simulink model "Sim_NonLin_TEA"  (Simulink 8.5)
settings: Solver=ode113  StartTime=0.0  StopTime=97200  RelTol=1e-3
InitFcn:
  | start
StopFcn:
  | Pl3
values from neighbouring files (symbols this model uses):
  Ave = [    [vehicle_flex34.m]    (also in vehicle_rigid.m)
  Bve = [    [vehicle_flex34.m]    (also in vehicle_rigid.m)
  CB2L = [cpsi, -cphi*spsi,  sphi*spsi;          0,    cphi,      -sphi;          0,    sphi*cpsi,  cphi*cpsi]/cpsi    [Rigbod_Dynam_LVLH.m]    (also in start.m = eye(3); start2.m = eye(3); start3.m = eye(3); start1.m = eye(3))
  Cve = [    [vehicle_flex34.m]    (also in vehicle_rigid.m)
  Dve = [    [vehicle_flex34.m]    (also in vehicle_rigid.m)
  ini = [wbo; atto; Hco]    [start.m]    (also in start2.m; start3.m; start1.m)
  Kpqr = lqr(sys,Q0,R0)    [des.m]
  nt = 12    [start.m]    (also in start2.m; start3.m; start1.m)
  wo = 0.0011    [start.m]    (also in start2.m; start3.m; start1.m)
undefined symbols (not defined in the file or in its folder): Rigbod_Dynam_LVLH

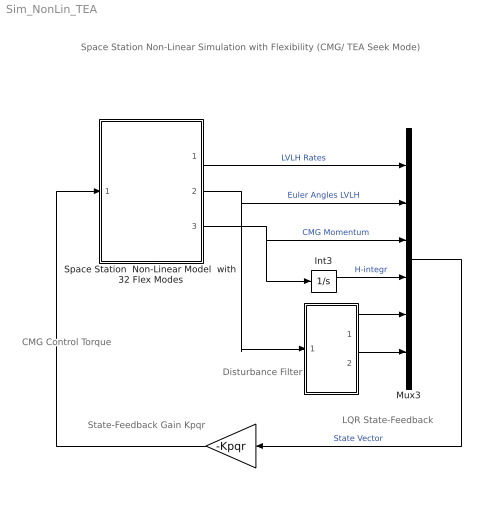
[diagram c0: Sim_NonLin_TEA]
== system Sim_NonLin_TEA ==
  note: Space Station Non-Linear Simulation with Flexibility (CMG/ TEA Seek Mode)
  note: LQR State-Feedback
  note: CMG Control Torque
  note: Disturbance Filter
  note: State-Feedback Gain Kpqr
  " " : Subsystem
  "  " : Gain  Gain=-Kpqr  Multiplication=Matrix(K*u)
  Int3 : Integrator
  Mux3 : Mux  Inputs=[3, 3, 3, 3, 1, 1]
  Space Station  Non-Linear Model  with 32 Flex Modes : Subsystem
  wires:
  Int3/1 -> Mux3/4  "H-integr"
  Space Station  Non-Linear Model  with 32 Flex Modes/3(Hcmg) -> Int3/1, Mux3/3  "CMG Momentum"
  Space Station  Non-Linear Model  with 32 Flex Modes/2(attit-lv) -> Mux3/2, " "/1(the)  "Euler Angles LVLH"
  "  "/1 -> Space Station  Non-Linear Model  with 32 Flex Modes/1(Tcmg)
  Mux3/1 -> "  "/1  "State Vector"
  " "/1(a1) -> Mux3/5
  " "/2(a2) -> Mux3/6
  Space Station  Non-Linear Model  with 32 Flex Modes/1(w-lv) -> Mux3/1  "LVLH Rates"

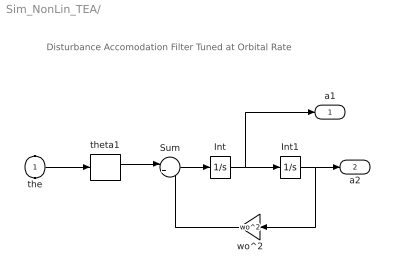
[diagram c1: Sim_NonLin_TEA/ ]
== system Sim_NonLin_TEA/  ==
  note: Disturbance Accomodation Filter Tuned at Orbital Rate
  the : Inport
  Int : Integrator
  Int1 : Integrator
  Sum : Sum  Inputs=|+-
  theta1 : Selector  InputPortWidth=3  Indices=[2]
  wo^2 : Gain  Gain=wo^2
  a1 : Outport
  a2 : Outport  Port=2
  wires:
  Int/1 -> Int1/1, a1/1
  Sum/1 -> Int/1
  Int1/1 -> wo^2/1, a2/1
  wo^2/1 -> Sum/2
  theta1/1 -> Sum/1
  the/1 -> theta1/1

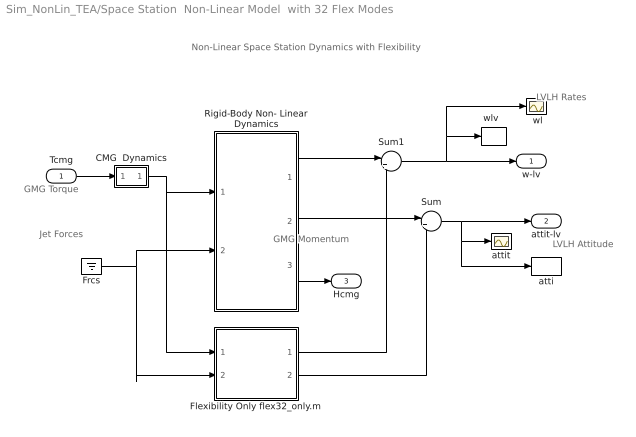
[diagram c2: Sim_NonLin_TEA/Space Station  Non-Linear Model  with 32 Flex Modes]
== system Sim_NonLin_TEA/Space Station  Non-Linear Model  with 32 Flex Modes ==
  note: Non-Linear Space Station Dynamics with Flexibility
  note: GMG Torque
  note: Jet Forces
  note: LVLH Rates
  note: LVLH Attitude
  note: GMG Momentum
  Tcmg : Inport
  " attit " : Scope
  " wl" : Scope
  CMG  Dynamics : Subsystem
  Flexibility Only flex32_only.m : Subsystem
  Frcs : Ground
  Rigid-Body Non- Linear Dynamics : Subsystem
  Sum : Sum  Inputs=|++
  Sum1 : Sum  Inputs=|++
  atti : ToWorkspace  VariableName=theta  SampleTime=-1
  "wlv  " : ToWorkspace  VariableName=wl  SampleTime=-1
  w-lv : Outport
  attit-lv : Outport  Port=2
  Hcmg : Outport  Port=3
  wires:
  Frcs/1 -> Rigid-Body Non- Linear Dynamics/2(Frcs), Flexibility Only flex32_only.m/2(Frcs)
  Rigid-Body Non- Linear Dynamics/2(atti-lv) -> Sum/1
  Flexibility Only flex32_only.m/2(att) -> Sum/2
  Sum/1 -> attit-lv/1, " attit "/1, atti/1
  Sum1/1 -> w-lv/1, "wlv  "/1, " wl"/1
  Tcmg/1 -> CMG  Dynamics/1(I)
  Rigid-Body Non- Linear Dynamics/1(w-lv) -> Sum1/1
  Flexibility Only flex32_only.m/1(wbf) -> Sum1/2
  Rigid-Body Non- Linear Dynamics/3(Hcmg) -> Hcmg/1
  CMG  Dynamics/1(O) -> Rigid-Body Non- Linear Dynamics/1(Tcmg), Flexibility Only flex32_only.m/1(Tcmg)

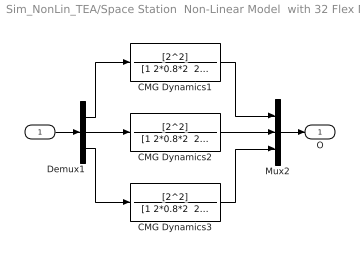
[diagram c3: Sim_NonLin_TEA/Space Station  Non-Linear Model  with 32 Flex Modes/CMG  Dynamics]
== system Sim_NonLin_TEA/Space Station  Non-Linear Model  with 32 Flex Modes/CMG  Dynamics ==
  I : Inport
  CMG Dynamics1 : TransferFcn  Numerator=[2^2]  Denominator="[1 2*0.8*2  2^2]"
  CMG Dynamics2 : TransferFcn  Numerator=[2^2]  Denominator="[1 2*0.8*2  2^2]"
  CMG Dynamics3 : TransferFcn  Numerator=[2^2]  Denominator="[1 2*0.8*2  2^2]"
  Demux1 : Demux  Outputs=3
  Mux2 : Mux  Inputs=3
  O : Outport
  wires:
  Mux2/1 -> O/1
  I/1 -> Demux1/1
  Demux1/3 -> CMG Dynamics3/1
  Demux1/1 -> CMG Dynamics1/1
  Demux1/2 -> CMG Dynamics2/1
  CMG Dynamics1/1 -> Mux2/1
  CMG Dynamics3/1 -> Mux2/3
  CMG Dynamics2/1 -> Mux2/2

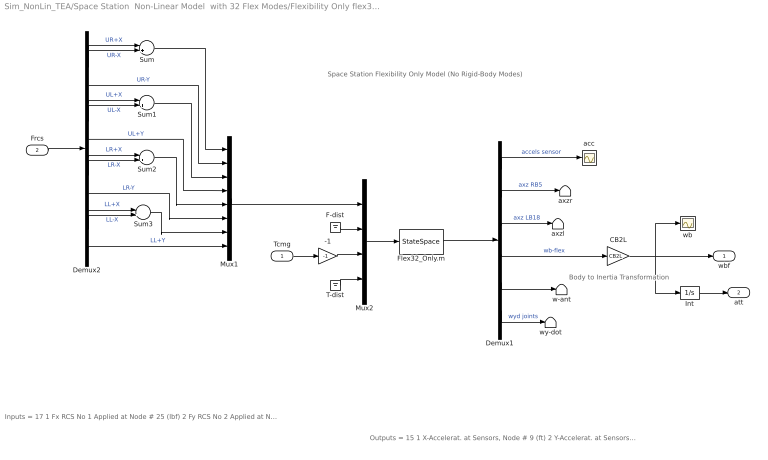
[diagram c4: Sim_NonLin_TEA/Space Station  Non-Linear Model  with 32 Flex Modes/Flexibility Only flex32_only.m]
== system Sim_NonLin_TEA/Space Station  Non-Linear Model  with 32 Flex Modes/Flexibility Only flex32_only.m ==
  note: Outputs = 15 1 X-Accelerat. at Sensors, Node # 9 (ft) 2 Y-Accelerat. at Sensors, Node # 9 (ft) 3 Z-Accelerat. at Sensors, Node # 9 (ft) 4 X-Accelerat. at Right Boom End, Node # 5 (ft) 5 Z-Accelerat. at Right Boom End, Node # 5 (ft) 6 X-Accelerat. at Left Boom End, Node # 18 (ft) 7 Z-Accelerat. at Left Boom End, Node # 18 (ft) 8 X-Rot. Rate at Sensors, Node # 9 (radian) 9 Y-Rot. Rate at Sensors, Node # 9 (radian) 10 Z-Rot. Rate at Sensors, Node # 9 (radian) 11 X-Rot. Rate at Antena Bot-Left, Node # 24 (radian) 12 Y-Rot. Rate at Antena Bot-Left, Node # 24 (radian) 13 Z-Rot. Rate at Antena Bot-Left, Node # 24 (radian) 14 Y-Rot.Accel. at Right Joint, Node # 7 (radian) 15 Y-Rot.Accel. at Left Joint, Node # 16 (radian)
  note: Inputs = 17 1 Fx RCS No 1 Applied at Node # 25 (lbf) 2 Fy RCS No 2 Applied at Node # 25 (lbf) 3 Fx RCS No 3 Applied at Node # 26 (lbf) 4 Fy RCS No 4 Applied at Node # 26 (lbf) 5 Fx RCS No 5 Applied at Node # 27 (lbf) 6 Fy RCS No 6 Applied at Node # 27 (lbf) 7 Fx RCS No 7 Applied at Node # 28 (lbf) 8 Fy RCS No 8 Applied at Node # 28 (lbf) 9 Fx Disturb. No 9 at Node # 21 (lbf) 10 Fy Disturb. No 10 at Node # 21 (lbf) 11 Fz Disturb. No 11 at Node # 21 (lbf) 12 Torq-x No 1 CMG Applied at Node # 10 (ft-lb) 13 Torq-y No 2 CMG Applied at Node # 10 (ft-lb) 14 Torq-z No 3 CMG Applied at Node # 10 (ft-lb) 15 Torq-x No 4 Gimbal Dist. at Node # 1 (ft-lb) 16 Torq-y No 5 Gimbal Dist. at Node # 1 (ft-lb) 17 Torq-z No 6 Gimbal Dist. at Node # 1 (ft-lb)
  note: Space Station Flexibility Only Model (No Rigid-Body Modes)
  note: Body to Inertia Transformation
  Tcmg : Inport
  Frcs : Inport  Port=2
  -1 : Gain  Gain=-1
  CB2L : Gain  Gain=CB2L  Multiplication=Matrix(K*u)
  Demux1 : Demux  Outputs=[3, 2, 2, 3, 3, 2]
  Demux2 : Demux  Outputs=12
  F-dist : Ground
  Flex32_Only.m : StateSpace  A=Ave  B=Bve  C=Cve  D=Dve  X0=0
  Int : Integrator
  Mux1 : Mux  Inputs=8
  Mux2 : Mux  Inputs=[8, 3, 3, 3]
  Sum{,1..3} (4 alike) : Sum  Inputs=|+-
  T-dist : Ground
  acc : Scope
  axzl : Terminator
  axzr : Terminator
  w-ant : Terminator
  wb : Scope
  wy-dot : Terminator
  wbf : Outport
  att : Outport  Port=2
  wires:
  Demux1/6 -> wy-dot/1  "wyd joints"
  Demux1/5 -> w-ant/1
  T-dist/1 -> Mux2/4
  F-dist/1 -> Mux2/2
  Demux1/3 -> axzl/1  "axz LB18"
  Demux1/2 -> axzr/1  "axz RB5"
  Tcmg/1 -> -1/1
  Demux1/4 -> CB2L/1  "wb-flex"
  Demux1/1 -> acc/1  "accels sensor"
  Flex32_Only.m/1 -> Demux1/1
  Mux2/1 -> Flex32_Only.m/1
  Mux1/1 -> Mux2/1
  Frcs/1 -> Demux2/1
  Demux2/6 -> Mux1/4  "UL+Y"
  Demux2/9 -> Mux1/6  "LR-Y"
  Demux2/12 -> Mux1/8  "LL+Y"
  Demux2/3 -> Mux1/2  "UR-Y"
  Demux2/1 -> Sum/1  "UR+X"
  Demux2/2 -> Sum/2  "UR-X"
  Sum/1 -> Mux1/1
  Demux2/4 -> Sum1/1  "UL+X"
  Demux2/5 -> Sum1/2  "UL-X"
  Sum1/1 -> Mux1/3
  Demux2/7 -> Sum2/1  "LR+X"
  Demux2/8 -> Sum2/2  "LR-X"
  Demux2/10 -> Sum3/1  "LL+X"
  Demux2/11 -> Sum3/2  "LL-X"
  Sum3/1 -> Mux1/7
  Sum2/1 -> Mux1/5
  Int/1 -> att/1
  -1/1 -> Mux2/3
  CB2L/1 -> wb/1, wbf/1, Int/1

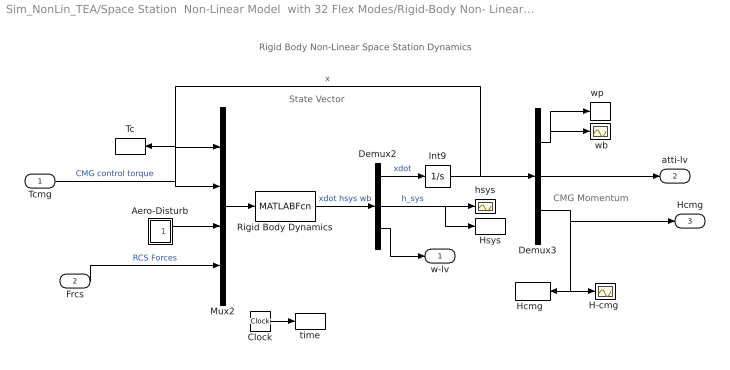
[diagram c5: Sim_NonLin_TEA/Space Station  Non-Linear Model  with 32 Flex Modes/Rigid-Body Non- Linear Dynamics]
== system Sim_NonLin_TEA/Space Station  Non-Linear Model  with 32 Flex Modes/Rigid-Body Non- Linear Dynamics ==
  note: CMG Momentum
  note: State Vector
  note: Rigid Body Non-Linear Space Station Dynamics
  Tcmg : Inport  PortDimensions=3
  Frcs : Inport  Port=2  PortDimensions=nt
  " wb" : Scope
  Aero-Disturb : Subsystem
  Clock : Clock
  Demux2 : Demux  Outputs=[9,3,3]
  Demux3 : Demux  Outputs=[3,3,3]
  "H-cmg " : Scope
  "Hcmg  " : ToWorkspace  VariableName=Hcmg  SampleTime=-1
  Hsys : ToWorkspace  VariableName=Hsys  SampleTime=-1
  Int9 : Integrator  InitialCondition=ini
  Mux2 : Mux  Inputs=[9, 3, 3, nt]
  Rigid Body Dynamics : MATLABFcn  MATLABFcn=Rigbod_Dynam_LVLH( u(1:9), u(10:12), u(13:15), u(16:15+nt) )  OutputDimensions=15
  Tc : ToWorkspace  VariableName=Tcmg  SampleTime=-1
  hsys : Scope
  time : ToWorkspace  VariableName=time  SampleTime=-1
  "wp  " : ToWorkspace  VariableName=wb  SampleTime=-1
  w-lv : Outport
  atti-lv : Outport  Port=2
  Hcmg : Outport  Port=3
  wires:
  Mux2/1 -> Rigid Body Dynamics/1
  Clock/1 -> time/1
  Frcs/1 -> Mux2/4  "RCS Forces"
  Demux3/3 -> Hcmg/1, "H-cmg "/1, "Hcmg  "/1
  Demux3/2 -> atti-lv/1
  Demux2/2 -> Hsys/1, hsys/1  "h_sys"
  Demux2/3 -> w-lv/1
  Tcmg/1 -> Mux2/2, Tc/1  "CMG control torque"
  Int9/1 -> Mux2/1, Demux3/1  "x"
  Demux2/1 -> Int9/1  "xdot"
  Rigid Body Dynamics/1 -> Demux2/1  "xdot hsys wb"
  Demux3/1 -> " wb"/1, "wp  "/1
  Aero-Disturb/1(Td) -> Mux2/3

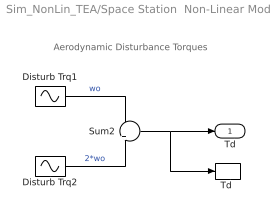
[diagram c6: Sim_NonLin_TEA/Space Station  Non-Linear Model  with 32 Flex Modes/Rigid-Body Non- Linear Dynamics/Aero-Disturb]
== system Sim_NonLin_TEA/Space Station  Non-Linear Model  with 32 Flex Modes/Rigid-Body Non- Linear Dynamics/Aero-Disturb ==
  note: Aerodynamic Disturbance Torques
  Disturb Trq1 : Sin  Amplitude=[1, 3, 1]  Bias="[1  8  1]"  Frequency=[wo, wo, wo]  SampleTime=0
  Disturb Trq2 : Sin  Amplitude=[1, 1, 1]*0.5  Frequency=[wo, wo, wo]*2  SampleTime=0
  Sum2 : Sum  Inputs=+|+
  "Td " : ToWorkspace  VariableName=Td  SampleTime=-1
  Td : Outport
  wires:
  Disturb Trq2/1 -> Sum2/2  "2*wo"
  Sum2/1 -> "Td "/1, Td/1
  Disturb Trq1/1 -> Sum2/1  "wo"
